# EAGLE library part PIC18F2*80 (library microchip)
28-Pin Enhanced Flash Microcontrollers with ECAN(TM) Technology 10-Bit A/D and nanoWatt Technology Source: http://www.microchip.com .. 39637a.pdf
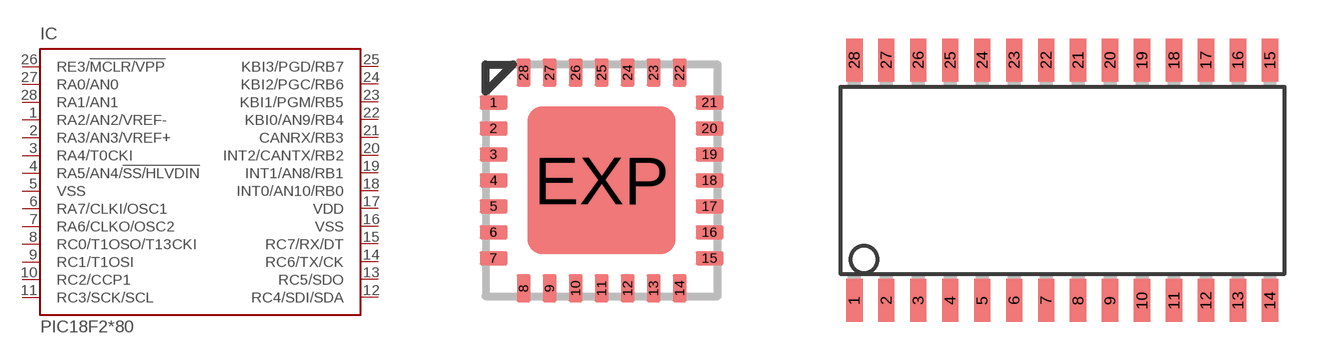
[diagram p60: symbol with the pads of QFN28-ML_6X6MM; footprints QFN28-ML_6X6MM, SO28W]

Designator prefix IC

## PIC18F2480-I/ML (MF: MICROCHIP; MPN: PIC18F2480-I/ML; OC_FARNELL: 1556179; OC_NEWARK: 71J7235), PIC18F2580-I/ML (MF: MICROCHIP; MPN: PIC18F2580-I/ML; OC_FARNELL: 1556180; OC_NEWARK: 71J7242)  [QFN28-ML_6X6MM]
1  RA2/AN2/VREF-
2  RA3/AN3/VREF+
3  RA4/T0CKI
4  RA5/AN4/!SS/HLVDIN
5  VSS  pwr
6  RA7/CLKI/OSC1  in
7  RA6/CLKO/OSC2  out
8  RC0/T1OSO/T13CKI
9  RC1/T1OSI
10  RC2/CCP1
11  RC3/SCK/SCL
12  RC4/SDI/SDA
13  RC5/SDO
14  RC6/TX/CK
15  RC7/RX/DT
16  VSS  pwr
17  VDD  pwr
18  INT0/AN10/RB0
19  INT1/AN8/RB1
20  INT2/CANTX/RB2
21  CANRX/RB3
22  KBI0/AN9/RB4
23  KBI1/PGM/RB5
24  KBI2/PGC/RB6
25  KBI3/PGD/RB7
26  RE3/!MCLR/VPP  in
27  RA0/AN0
28  RA1/AN1

## PIC18F2580-E/SO (MF: MICROCHIP; MPN: PIC18F2580-I/SO; OC_FARNELL: 9321284; OC_NEWARK: 71J7243)  [SO28W]
1  RE3/!MCLR/VPP  in
2  RA0/AN0
3  RA1/AN1
4  RA2/AN2/VREF-
5  RA3/AN3/VREF+
6  RA4/T0CKI
7  RA5/AN4/!SS/HLVDIN
8  VSS  pwr
9  RA7/CLKI/OSC1  in
10  RA6/CLKO/OSC2  out
11  RC0/T1OSO/T13CKI
12  RC1/T1OSI
13  RC2/CCP1
14  RC3/SCK/SCL
15  RC4/SDI/SDA
16  RC5/SDO
17  RC6/TX/CK
18  RC7/RX/DT
19  VSS  pwr
20  VDD  pwr
21  INT0/AN10/RB0
22  INT1/AN8/RB1
23  INT2/CANTX/RB2
24  CANRX/RB3
25  KBI0/AN9/RB4
26  KBI1/PGM/RB5
27  KBI2/PGC/RB6
28  KBI3/PGD/RB7

## PIC18F2480-I/SP (MF: MICROCHIP; MPN: PIC18F2480-I/SP; OC_FARNELL: 9321217; OC_NEWARK: 71J7237), PIC18F2580-I/SP (MF: MICROCHIP; MPN: PIC18F2580-I/SP; OC_FARNELL: 9321276; OC_NEWARK: 71J7244)  [DIL28-3]
Pads as for SO28W

## Footprint QFN28-ML_6X6MM (pad centres in mm)
QFN28-ML_6X6MM Source: http://www.microchip.com .. 39637a.pdf
smd 0.7 x 0.35: 1 -2.7,1.95; 2 -2.7,1.3; 3 -2.7,0.65; 4 -2.7,0; 5 -2.7,-0.65; 6 -2.7,-1.3; 7 -2.7,-1.95; 15 2.7,-1.95; 16 2.7,-1.3; 17 2.7,-0.65; 18 2.7,0; 19 2.7,0.65; 20 2.7,1.3; 21 2.7,1.95
smd 0.35 x 0.7: 8 -1.95,-2.7; 9 -1.3,-2.7; 10 -0.65,-2.7; 11 0,-2.7; 12 0.65,-2.7; 13 1.3,-2.7; 14 1.95,-2.7; 22 1.95,2.7; 23 1.3,2.7; 24 0.65,2.7; 25 0,2.7; 26 -0.65,2.7; 27 -1.3,2.7; 28 -1.95,2.7
smd 3.7 x 3.7: EXP 0,0

## Footprint SO28W (pad centres in mm)
28-Lead Plastic Small Outline (SO) Wide, 300 mil Body (SOIC) Source: http://ww1.microchip.com/downloads/en/devicedoc/39632c.pdf
smd 0.65 x 1.7: 1 -7.62,-4.78; 2 -6.35,-4.78; 3 -5.08,-4.78; 4 -3.81,-4.78; 5 -2.54,-4.78; 6 -1.27,-4.78; 7 0,-4.78; 8 1.27,-4.78; 9 2.54,-4.78; 10 3.81,-4.78; 11 5.08,-4.78; 12 6.35,-4.78; 13 7.62,-4.78; 14 8.89,-4.78; 15 8.89,4.78; 16 7.62,4.78; 17 6.35,4.78; 18 5.08,4.78; 19 3.81,4.78; 20 2.54,4.78; 21 1.27,4.78; 22 0,4.78; 23 -1.27,4.78; 24 -2.54,4.78; 25 -3.81,4.78; 26 -5.08,4.78; 27 -6.35,4.78; 28 -7.62,4.78

## Footprint DIL28-3 (pad centres in mm)
Dual In Line package type P
drill 0.813 long: 1 -16.51,-3.81; 2 -13.97,-3.81; 3 -11.43,-3.81; 4 -8.89,-3.81; 5 -6.35,-3.81; 6 -3.81,-3.81; 7 -1.27,-3.81; 8 1.27,-3.81; 9 3.81,-3.81; 10 6.35,-3.81; 11 8.89,-3.81; 12 11.43,-3.81; 13 13.97,-3.81; 14 16.51,-3.81; 15 16.51,3.81; 16 13.97,3.81; 17 11.43,3.81; 18 8.89,3.81; 19 6.35,3.81; 20 3.81,3.81; 21 1.27,3.81; 22 -1.27,3.81; 23 -3.81,3.81; 24 -6.35,3.81; 25 -8.89,3.81; 26 -11.43,3.81; 27 -13.97,3.81; 28 -16.51,3.81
